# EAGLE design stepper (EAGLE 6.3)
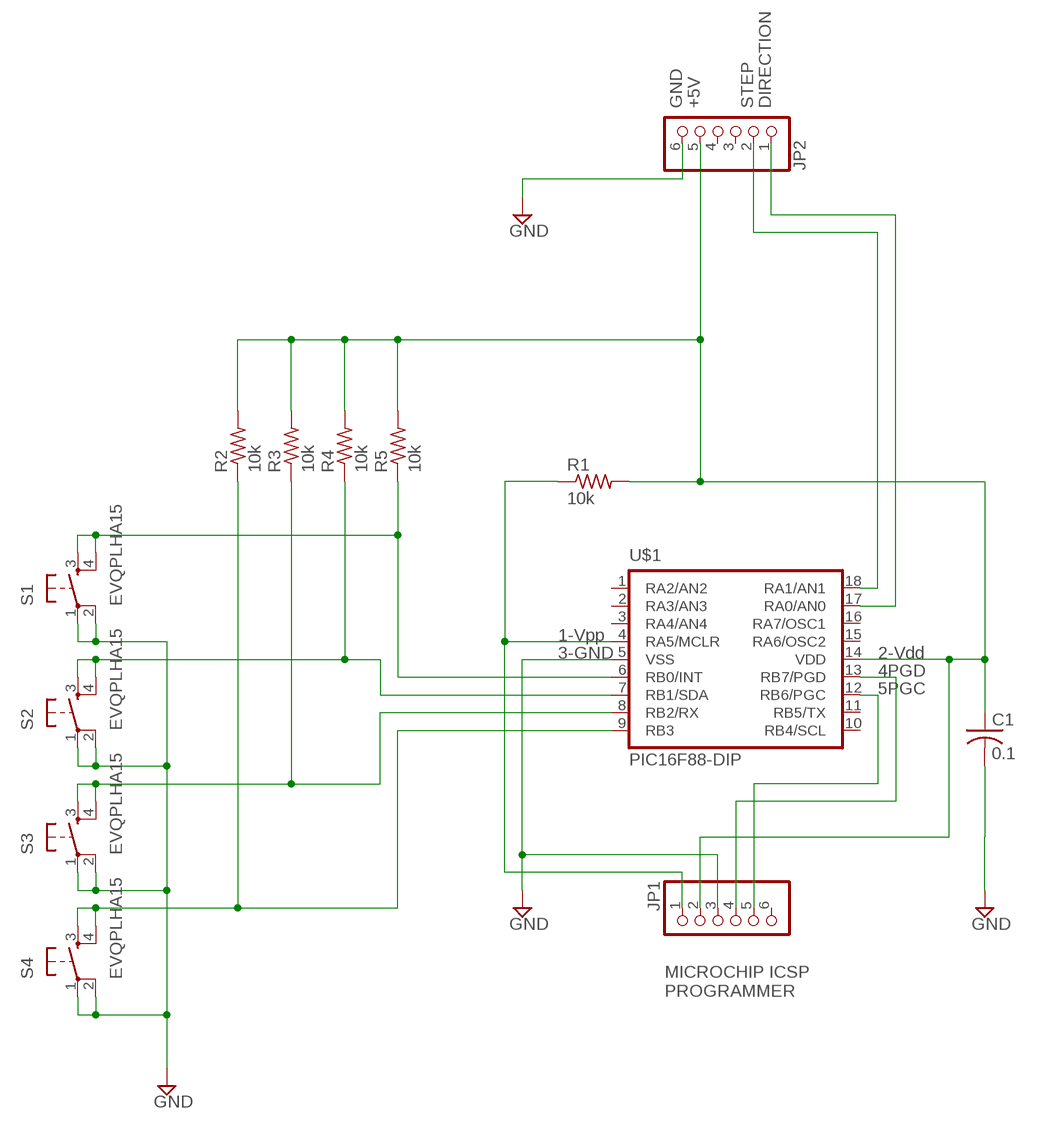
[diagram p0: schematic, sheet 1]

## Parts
C1  0.1  C-US025-025X050  [C025-025X050]
JP1  PINHD-1X6  [1X06]
JP2  PINHD-1X6  [1X06]
R1  10k  R-US_0207/9  [0207/9]
R2  10k  R-US_0207/9  [0207/9]
R3  10k  R-US_0207/9  [0207/9]
R4  10k  R-US_0207/9  [0207/9]
R5  10k  R-US_0207/9  [0207/9]
S1  EVQPLHA15  TAC_SWITCHSMD  [TACTILE_SWITCH_SMD]
S2  EVQPLHA15  TAC_SWITCHSMD  [TACTILE_SWITCH_SMD]
S3  EVQPLHA15  TAC_SWITCHSMD  [TACTILE_SWITCH_SMD]
S4  EVQPLHA15  TAC_SWITCHSMD  [TACTILE_SWITCH_SMD]
U$1  PIC16F88-DIP  [DIL18]

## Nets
GND: C1.2 JP1.3 JP2.6 S1.1 S1.2 S2.1 S2.2 S3.1 S3.2 S4.1 S4.2 U$1.5(VSS)
N$1: JP1.1 R1.1 U$1.4(RA5/MCLR)
N$4: JP1.4 U$1.13(RB7/PGD)
N$5: JP1.5 U$1.12(RB6/PGC)
N$6: JP2.2 U$1.18(RA1/AN1)
N$7: JP2.1 U$1.17(RA0/AN0)
N$8: C1.1 JP1.2 JP2.5 R1.2 R2.2 R3.2 R4.2 R5.2 U$1.14(VDD)
N$10: R5.1 S1.3 S1.4 U$1.6(RB0/INT)
N$11: R4.1 S2.3 S2.4 U$1.7(RB1/SDA)
N$12: R3.1 S3.3 S3.4 U$1.8(RB2/RX)
N$13: R2.1 S4.3 S4.4 U$1.9(RB3)
Unconnected: JP1.6 JP2.3 JP2.4 U$1.1(RA2/AN2) U$1.2(RA3/AN3) U$1.3(RA4/AN4) U$1.10(RB4/SCL) U$1.11(RB5/TX) U$1.15(RA6/OSC2) U$1.16(RA7/OSC1)

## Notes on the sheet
- GND | +5V | STEP | DIRECTION
- 1-Vpp
- 3-GND | 2-Vdd
- 4PGD
- 5PGC
- MICROCHIP ICSP
  PROGRAMMER

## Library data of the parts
C1 = adafruit:C-US: CAPACITOR, American symbol; MPN: FG16C0G1H104JNT06
JP1 JP2 = adafruit:PINHD-1X6: PIN HEADER
R1-R5 = adafruit:R-US_: RESISTOR, American symbol; MPN: MF1/4LCT52R103J
S1-S4 = SparkFun:TAC_SWITCH: Momentary Switch Button commonly used for reset or general input. Spark Fun Electronics SKU : COM-00097; MPN: EVQ-PLHA15
U$1 = SparkFun:PIC16F88-DIP; MPN: PIC16F88-I/P

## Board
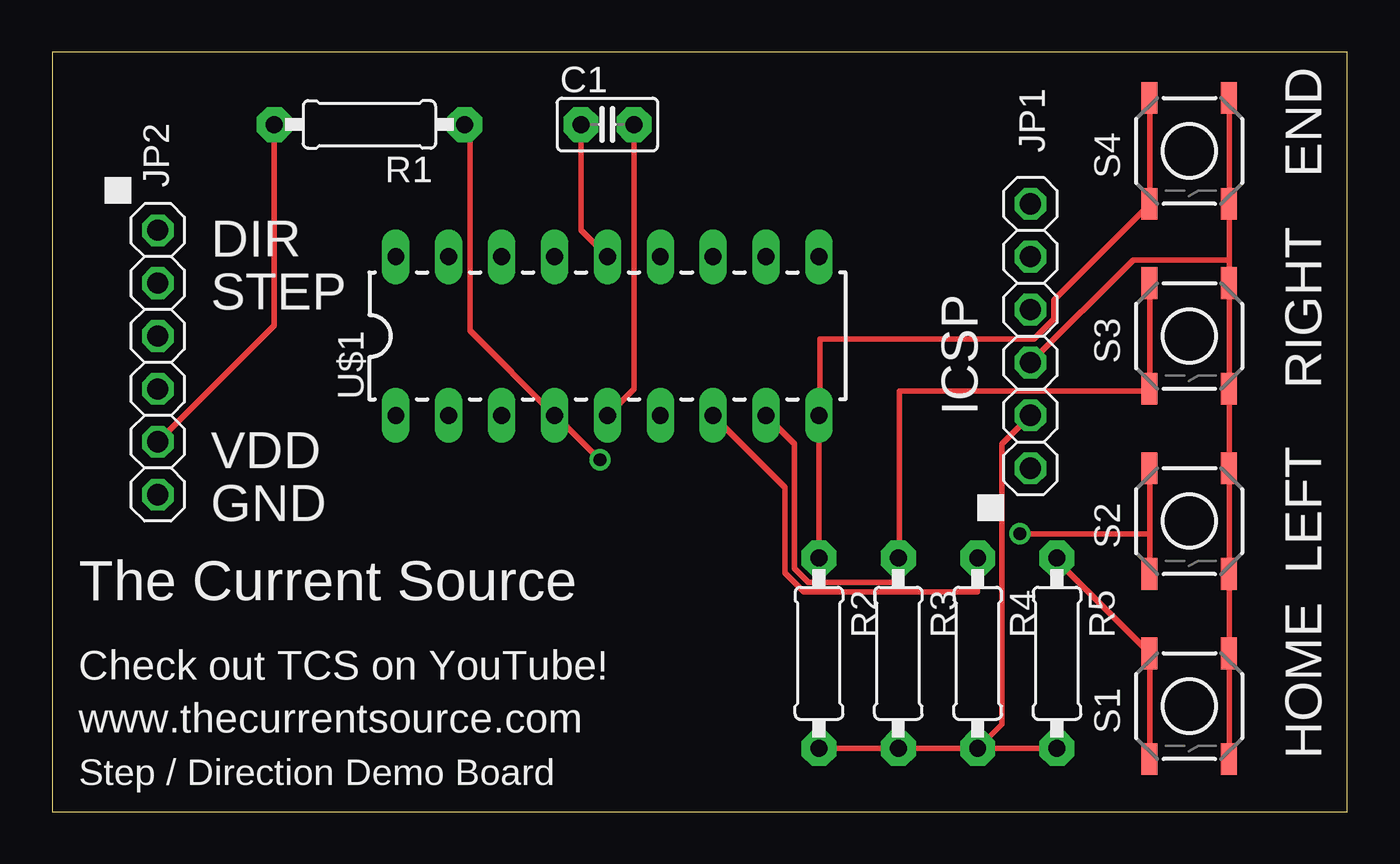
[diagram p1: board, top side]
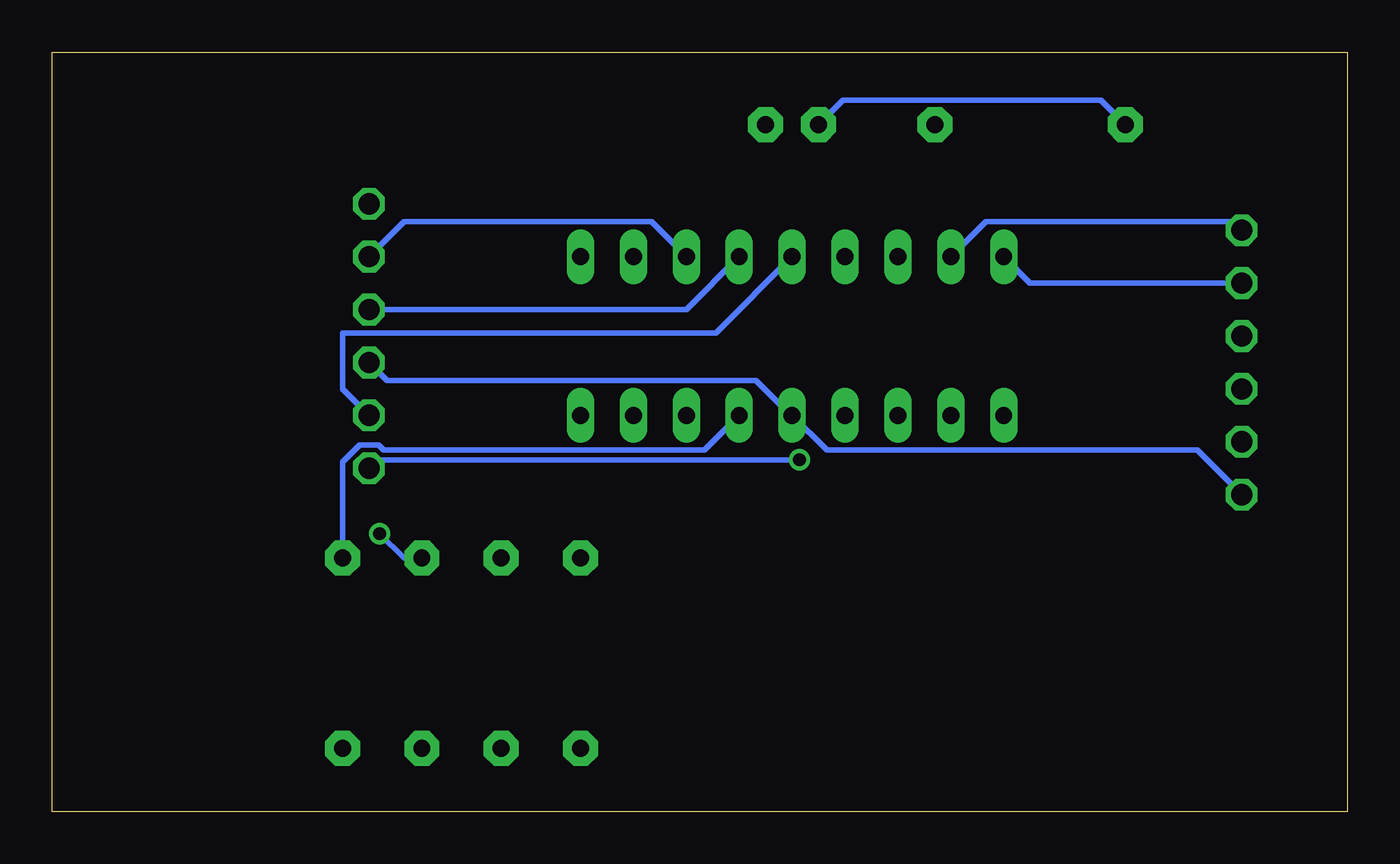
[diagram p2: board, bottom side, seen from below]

Size 62.21 x 36.5 mm. Coordinates in mm from the lower left corner, seen from the top.
Outline: 0,0 62.21,0 62.21,36.5 0,36.5 0,0
Copper layers (1*16): Top 0.035mm / dielectric 1.5mm / Bottom 0.035mm
Design rules "default": minimum track width 10mil, minimum drill 24mil, track to track 8mil, track to pad 8mil, pad to pad 8mil, via to via 8mil, smd to smd 8mil, copper to edge 40mil, drill to drill 8mil, minimum pad ring 10mil, minimum via ring 8mil, stop-mask expansion 4mil, vias tented up to drill 0mil, thermal gap 10mil

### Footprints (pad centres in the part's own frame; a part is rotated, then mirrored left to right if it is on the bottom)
C025-025X050 = drill 0.813 pad 1.676 octagon: 1 -1.27,0; 2 1.27,0
1X06 = drill 1.016 octagon: 1 -6.35,0; 2 -3.81,0; 3 -1.27,0; 4 1.27,0; 5 3.81,0; 6 6.35,0
0207/9 = drill 0.813 pad 1.676 octagon: 1 -4.572,0; 2 4.572,0
TACTILE_SWITCH_SMD = smd 1.524 x 0.762: 1 -2.54,1.905; 2 2.54,1.905; 3 -2.54,-1.905; 4 2.54,-1.905
DIL18 = drill 0.813 long: 1 -10.16,-3.81; 2 -7.62,-3.81; 3 -5.08,-3.81; 4 -2.54,-3.81; 5 0,-3.81; 6 2.54,-3.81; 7 5.08,-3.81; 8 7.62,-3.81; 9 10.16,-3.81; 10 10.16,3.81; 11 7.62,3.81; 12 5.08,3.81; 13 2.54,3.81; 14 0,3.81; 15 -2.54,3.81; 16 -5.08,3.81; 17 -7.62,3.81; 18 -10.16,3.81

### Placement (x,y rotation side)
C1  26.67,33.02 0 top
JP1  46.99,22.86 90 top
JP2  5.08,21.59 270 top
R1  15.24,33.02 180 top
R2  36.83,7.62 270 top
R3  40.64,7.62 270 top
R4  44.45,7.62 270 top
R5  48.26,7.62 270 top
S1  54.61,5.08 270 top
S2  54.61,13.97 270 top
S3  54.61,22.86 270 top
S4  54.61,31.75 270 top
U$1  26.67,22.86 0 top

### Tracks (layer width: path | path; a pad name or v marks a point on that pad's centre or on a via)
GND
  Top 0.254: S1.2 56.54,2.54 56.54,7.62 S1.1 56.54,7.72 56.54,11.43 S2.2 56.54,11.53 56.54,16.41 S2.1 56.54,16.51 56.54,20.32 S3.2 56.54,20.42 56.54,25.3 S3.1 56.54,25.4 56.54,26.52 | 56.54,26.52 56.54,29.21 S4.2 56.54,29.31 56.54,34.29 S4.1 | JP1.3 51.92,26.52 56.44,26.52 56.54,26.52 | U$1.5 27.94,20.32 C1.2
  Bottom 0.254: JP2.6 7.21,17.37 24.99,17.37 U$1.5 26.77,19.1 28.4,20.73 46.13,20.73 JP1.3
N$1  (via drill 0.61)
  Top 0.254: R1.1 20.07,32.77 20.07,23.11 U$1.4 24.23,19 v26.31,16.92
  Bottom 0.254: JP1.1 46.58,16.92 v26.31,16.92
N$4
  Bottom 0.254: U$1.13 31.75,24.13 JP1.4
N$5
  Bottom 0.254: U$1.12 33.43,28.35 45.31,28.35 JP1.5
N$6
  Bottom 0.254: U$1.18 15.24,25.4 JP2.2
N$7
  Bottom 0.254: U$1.17 17.37,28.35 5.49,28.35 JP2.1
N$8
  Top 0.254: R2.2 R3.2 40.74,3.05 44.35,3.05 R4.2 | JP1.2 45.62,17.68 45.62,4.22 R4.2 | R5.2 44.6,3.05 R4.2 | U$1.14 25.4,27.94 C1.1 | JP2.5 10.67,23.37 R1.2
  Bottom 0.254: C1.1 24.23,34.19 11.84,34.19 R1.2 | JP1.2 48.26,20.32 48.26,23.01 30.33,23.01 U$1.14
N$10
  Top 0.254: S1.4 52.73,2.54 52.73,7.62 S1.3 52.63,7.72 48.26,12.09 R5.1
  Bottom 0.254: U$1.6 30.89,17.37 46.28,17.37 46.53,17.63 47.45,17.63 48.26,16.82 R5.1
N$11  (via drill 0.61)
  Top 0.254: 52.73,13.36 52.73,16.51 S2.3 | 52.73,13.36 52.73,11.43 S2.4 | U$1.7 35.2,15.6 35.2,11.48 36.12,10.57 44.45,10.57 R4.1 | v46.48,13.36 52.63,13.36 52.73,13.36
  Bottom 0.254: v46.48,13.36 45.31,12.19 R4.1
N$12
  Top 0.254: S3.3 52.73,25.4 52.73,20.32 S3.4 52.63,20.22 40.69,20.22 40.69,12.29 R3.1 40.64,11.02 36.32,11.02 35.66,11.68 35.66,17.68 U$1.8
N$13
  Top 0.254: S4.3 52.73,34.29 52.73,29.21 S4.4 52.63,29.11 48.11,24.59 48.11,23.67 47.14,22.71 36.88,22.71 36.88,19.15 U$1.9 R2.1

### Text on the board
_tsilk: END | DIR | STEP | RIGHT | ICSP | VDD | GND | LEFT | The Current Source | Check out TCS on YouTube! | www.thecurrentsource.com | HOME | Step / Direction Demo Board

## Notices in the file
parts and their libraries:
SparkFun: Licensing: CC v3.0 Share-Alike You are welcome to use this library for commercial purposes.
